| IBIS file stm32l4p5_4q5_ufqfpn48.ibs
[IBIS ver]   4.2
[File name]  stm32l4p5_4q5_ufqfpn48.ibs
[File Rev]   1.0
[Date]   26-12-2019
[Source]   Data Created at STMicroelectronics
[Notes]   File originated from ELDO simulations.
[Disclaimer] This information is for modeling purpose only and is
   not guaranted.
   The information is subject to change without notice.
[Copyright]  Copyright 2019 STMicroelectronics Inc.
|   Component stm32l4p5_4q5_ufqfpn48
[Component] stm32l4p5_4q5_ufqfpn48
[Manufacturer] STMicroelectronics
[Package]
| variable   typ   min   max
R_pkg  0  NA  NA
L_pkg  0  NA  NA
C_pkg  0  NA  NA
[Pin]   signal_name   model_name R_pin L_pin C_pin
1 VBAT POWER
2 PC13 io8prog2m25m50m120m_sudq_ft
3 PC14-OSC32_IN io8prog2m25m50m120m_sudq_ft
4 PC15-OSC32_OUT io8prog2m25m50m120m_sudq_ft
5 PH0-OSC_IN io8prog2m25m50m120m_sudq_ft
6 PH1-OSC_OUT io8prog2m25m50m120m_sudq_ft
7 NRST ioreset_ft_v33
8 VSSA GND
9 VDDA POWER
10 PA0 io8prog2m25m50m120m_sudq_ft
11 PA1 io8prog2m25m50m120m_sudq_ft
12 PA2 io8prog2m25m50m120m_sudq_ft
13 PA3 io8prog2m25m50m120m_sudq_ft
14 PA4 io8prog2m25m50m120m_sudq_ft
15 PA5 io8prog2m25m50m120m_sudq_ft
16 PA6 io8prog2m25m50m120m_sudq_ft
17 PA7 io8prog2m25m50m120m_sudq_ft
18 PB0 io8prog2m25m50m120m_sudq_ft
19 PB1 io8prog2m25m50m120m_sudq_ft
20 PB2 io8prog2m25m50m120m_sudq_ft
21 PB10 io8prog2m25m50m120m_sudq_i2c_ft
22 PB11 io8prog2m25m50m120m_sudq_i2c_ft
23 VSS GND
24 VDD POWER
25 PB12 io8w_swp_lcd4_ft
26 PB13 io8prog2m25m50m120m_sudq_i2c_ft
27 PB14 io8prog2m25m50m120m_sudq_i2c_ft
28 PB15 io8prog2m25m50m120m_sudq_ft
29 PA8 io8prog2m25m50m120m_sudq_ft
30 PA9 POWER
31 PA10 io8usb_id_otg20_lcd4_ft_ms
32 PA11 io8usblsfs_otg2
33 PA12 io8usblsfs_otg2
34 PA13 io8prog2m25m50m120m_sudq_ft
35 VSS GND
36 VDDUSB POWER
37 PA14 io8prog2m25m50m120m_sudq_ft
38 PA15 io8prog2m25m50m120m_sudq_ft
39 PB3 io8prog2m25m50m120m_sudq_ft
40 PB4 io8prog2m25m50m120m_sudq_ft
41 PB5 io8prog2m25m50m120m_sudq_ft
42 PB6 io8prog2m25m50m120m_sudq_i2c_ft
43 PB7 io8prog2m25m50m120m_sudq_i2c_ft
44 PH3-BOOT0 io8prog2m25m50m120m_sudq_ft
45 PB8 io8prog2m25m50m120m_sudq_i2c_ft
46 PB9 io8prog2m25m50m120m_sudq_i2c_ft
47 VSS GND
48 VDD POWER
[Model Selector] io8prog2m25m50m120m_sudq_ft
iols8p_sudq_ft_pd_lv  "IO low speed, PD=40kOhm - 1P8V"
iols8p_sudq_ft_pu_lv  "IO low speed, PU=40kOhm - 1P8V"
iols8p_sudq_ft_lv  "IO low speed - 1P8V"
iols8p_sudq_ft_pd  "IO low speed, PD=40kOhm - 3P3V"
iols8p_sudq_ft_pu  "IO low speed, PU=40kOhm - 3P3V"
iols8p_sudq_ft  "IO low speed - 3P3V"
iofs8p_sudq_ft_pd_lv  "IO full speed, PD=40kOhm - 1P8V"
iofs8p_sudq_ft_pu_lv  "IO full speed, PU=40kOhm - 1P8V"
iofs8p_sudq_ft_lv  "IO full speed - 1P8V"
iofs8p_sudq_ft_pd  "IO full speed, PD=40kOhm - 3P3V"
iofs8p_sudq_ft_pu  "IO full speed, PU=40kOhm - 3P3V"
iofs8p_sudq_ft  "IO full speed - 3P3V"
ioms8p_sudq_ft_pd_lv  "IO medium speed, PD=40kOhm - 1P8V"
ioms8p_sudq_ft_pu_lv  "IO medium speed, PU=40kOhm - 1P8V"
ioms8p_sudq_ft_lv  "IO medium speed - 1P8V"
ioms8p_sudq_ft_pd  "IO medium speed, PD=40kOhm - 3P3V"
ioms8p_sudq_ft_pu  "IO medium speed, PU=40kOhm - 3P3V"
ioms8p_sudq_ft  "IO medium speed - 3P3V"
iohs8p_sudq_ft_pd_lv  "IO high speed, PD=40kOhm - 1P8V"
iohs8p_sudq_ft_pu_lv  "IO high speed, PU=40kOhm - 1P8V"
iohs8p_sudq_ft_lv  "IO high speed - 1P8V"
iohs8p_sudq_ft_pd  "IO high speed, PD=40kOhm - 3P3V"
iohs8p_sudq_ft_pu  "IO high speed, PU=40kOhm - 3P3V"
iohs8p_sudq_ft  "IO high speed - 3P3V"
[Model Selector] io8prog2m25m50m120m_sudq_i2c_ft
io8prog_1v8_i2c_pd  "5V Tol GPIO 1.8V range i2c functionality with pull down"
io8prog_1v8_i2c_pu  "5V Tol GPIO 1.8V range i2c functionality with pull up"
io8prog_1v8_i2c  "5V Tol GPIO 1.8V range i2c functionality"
io8prog_3v3_i2c_pd  "5V Tol GPIO 3.3V range i2c functionality with pull down"
io8prog_3v3_i2c_pu  "5V Tol GPIO 3.3V range i2c functionality with pull up"
io8prog_3v3_i2c  "5V Tol GPIO 3.3V range i2c functionality"
iols8p_sudq_ft_pd_lv  "IO low speed, PD=40kOhm - 1P8V"
iols8p_sudq_ft_pu_lv  "IO low speed, PU=40kOhm - 1P8V"
iols8p_sudq_ft_lv  "IO low speed - 1P8V"
iols8p_sudq_ft_pd  "IO low speed, PD=40kOhm - 3P3V"
iols8p_sudq_ft_pu  "IO low speed, PU=40kOhm - 3P3V"
iols8p_sudq_ft  "IO low speed - 3P3V"
iofs8p_sudq_ft_pd_lv  "IO full speed, PD=40kOhm - 1P8V"
iofs8p_sudq_ft_pu_lv  "IO full speed, PU=40kOhm - 1P8V"
iofs8p_sudq_ft_lv  "IO full speed - 1P8V"
iofs8p_sudq_ft_pd  "IO full speed, PD=40kOhm - 3P3V"
iofs8p_sudq_ft_pu  "IO full speed, PU=40kOhm - 3P3V"
iofs8p_sudq_ft  "IO full speed - 3P3V"
ioms8p_sudq_ft_pd_lv  "IO medium speed, PD=40kOhm - 1P8V"
ioms8p_sudq_ft_pu_lv  "IO medium speed, PU=40kOhm - 1P8V"
ioms8p_sudq_ft_lv  "IO medium speed - 1P8V"
ioms8p_sudq_ft_pd  "IO medium speed, PD=40kOhm - 3P3V"
ioms8p_sudq_ft_pu  "IO medium speed, PU=40kOhm - 3P3V"
ioms8p_sudq_ft  "IO medium speed - 3P3V"
iohs8p_sudq_ft_pd_lv  "IO high speed, PD=40kOhm - 1P8V"
iohs8p_sudq_ft_pu_lv  "IO high speed, PU=40kOhm - 1P8V"
iohs8p_sudq_ft_lv  "IO high speed - 1P8V"
iohs8p_sudq_ft_pd  "IO high speed, PD=40kOhm - 3P3V"
iohs8p_sudq_ft_pu  "IO high speed, PU=40kOhm - 3P3V"
iohs8p_sudq_ft  "IO high speed - 3P3V"
[Model Selector] io8w_swp_lcd4_ft
io8w_swp_classc  "Class C swp functionality"
io8w_swp_classb  "Class B swp functionality"
io8lsw_1v8_pd  "GPIO 1.8V range with pd io low speed"
io8lsw_1v8_pu  "GPIO 1.8V range with pu io low speed"
io8lsw_1v8  "GPIO 1.8V range io low speed"
io8lsw_3v3_pd  "GPIO 3.3V range with pd io low speed"
io8lsw_3v3_pu  "GPIO 3.3V range with pu io low speed"
io8lsw_3v3  "GPIO 3.3V range io low speed"
io8fsw_1v8_pd  "GPIO 1.8V range with pd io full speed"
io8fsw_1v8_pu  "GPIO 1.8V range with pu io full speed"
io8fsw_1v8  "GPIO 1.8V range io full speed"
io8fsw_3v3_pd  "GPIO 3.3V range with pd io full speed"
io8fsw_3v3_pu  "GPIO 3.3V range with pu io full speed"
io8fsw_3v3  "GPIO 3.3V range io full speed"
io8msw_1v8_pd  "GPIO 1.8V range with pd io medium speed"
io8msw_1v8_pu  "GPIO 1.8V range with pu io medium speed"
io8msw_1v8  "GPIO 1.8V range io medium speed"
io8msw_3v3_pd  "GPIO 3.3V range with pd io medium speed"
io8msw_3v3_pu  "GPIO 3.3V range with pu io medium speed"
io8msw_3v3  "GPIO 3.3V range io medium speed"
io8hsw_1v8_pd  "GPIO 1.8V range with pd io high speed"
io8hsw_1v8_pu  "GPIO 1.8V range with pu io high speed"
io8hsw_1v8  "GPIO 1.8V range io high speed"
io8hsw_3v3_pd  "GPIO 3.3V range with pd io high speed"
io8hsw_3v3_pu  "GPIO 3.3V range with pu io high speed"
io8hsw_3v3  "GPIO 3.3V range io high speed"
[Model Selector] io8usblsfs_otg2
usb_ls_pd  "USB Low Speed mode - Pull Down"
usb_ls_pu2  "USB Low Speed mode - Pull up 2"
usb_ls_pu  "USB Low Speed mode - Pull up"
usb_fs  "USB Low Speed mode"
usb_fs_pd  "USB Full Speed mode - Pull Down"
usb_fs_pu2  "USB Full Speed mode - Pull up 2"
usb_fs_pu  "USB Full Speed mode - Pull up"
[Model Selector] io8usb_id_otg20_lcd4_ft_ms
io8usbid_1v8_id_pu  "ID 1V8 range with pull up"
io8usbid_3v3_id_pu  "ID 3V3 range with pull up"
io8usbid_1v8_id  "ID 1V8 range"
io8usbid_3v3_id  "ID 3V3 range"
io8lsusbid_1v8_pd  "GPIO 1.8V range with pd io low speed"
io8lsusbid_1v8_pu  "GPIO 1.8V range with pu io low speed"
io8lsusbid_1v8  "GPIO 1.8V range io low speed"
io8lsusbid_3v3_pd  "GPIO 3.3V range with pd io low speed"
io8lsusbid_3v3_pu  "GPIO 3.3V range with pu io low speed"
io8lsusbid_3v3  "GPIO 3.3V range io low speed"
io8fsusbid_1v8_pd  "GPIO 1.8V range with pd io full speed"
io8fsusbid_1v8_pu  "GPIO 1.8V range with pu io full speed"
io8fsusbid_1v8  "GPIO 1.8V range io full speed"
io8fsusbid_3v3_pd  "GPIO 3.3V range with pd io full speed"
io8fsusbid_3v3_pu  "GPIO 3.3V range with pu io full speed"
io8fsusbid_3v3  "GPIO 3.3V range io full speed"
io8msusbid_1v8_pd  "GPIO 1.8V range with pd io medium speed"
io8msusbid_1v8_pu  "GPIO 1.8V range with pu io medium speed"
io8msusbid_1v8  "GPIO 1.8V range io medium speed"
io8msusbid_3v3_pd  "GPIO 3.3V range with pd io medium speed"
io8msusbid_3v3_pu  "GPIO 3.3V range with pu io medium speed"
io8msusbid_3v3  "GPIO 3.3V range io medium speed"
io8hsusbid_1v8_pd  "GPIO 1.8V range with pd io high speed"
io8hsusbid_1v8_pu  "GPIO 1.8V range with pu io high speed"
io8hsusbid_1v8  "GPIO 1.8V range io high speed"
io8hsusbid_3v3_pd  "GPIO 3.3V range with pd io high speed"
io8hsusbid_3v3_pu  "GPIO 3.3V range with pu io high speed"
io8hsusbid_3v3  "GPIO 3.3V range io high speed"
[Model Selector] ioreset_ft_v33
ioreset_1v2_pu  "RESET 1.2V range with PU"
ioreset_1v2  "RESET 1.2V range"
ioreset_1v8_pu  "RESET 1.8V range with PU"
ioreset_1v8  "RESET 1.8V range"
ioreset_3v3_pu  "RESET 3.3V range with PU"
ioreset_3v3  "RESET 3.3V range"
| Models and submodels in the file (97): iols8p_sudq_ft_pd_lv (I/O), iols8p_sudq_ft_pu_lv (I/O), iols8p_sudq_ft_lv (I/O), iols8p_sudq_ft_pd (I/O), iols8p_sudq_ft_pu (I/O), iols8p_sudq_ft (I/O), iofs8p_sudq_ft_pd_lv (I/O), iofs8p_sudq_ft_pu_lv (I/O), iofs8p_sudq_ft_lv (I/O), iofs8p_sudq_ft_pd (I/O), iofs8p_sudq_ft_pu (I/O), iofs8p_sudq_ft (I/O), ioms8p_sudq_ft_pd_lv (I/O), ioms8p_sudq_ft_pu_lv (I/O), ioms8p_sudq_ft_lv (I/O), ioms8p_sudq_ft_pd (I/O), ioms8p_sudq_ft_pu (I/O), ioms8p_sudq_ft (I/O), iohs8p_sudq_ft_pd_lv (I/O), iohs8p_sudq_ft_pu_lv (I/O), iohs8p_sudq_ft_lv (I/O), iohs8p_sudq_ft_pd (I/O), iohs8p_sudq_ft_pu (I/O), iohs8p_sudq_ft (I/O), io8prog_1v8_i2c_pd (I/O_open_drain), io8prog_1v8_i2c_pu (I/O_open_drain), io8prog_1v8_i2c (I/O_open_drain), io8prog_3v3_i2c_pd (I/O_open_drain), io8prog_3v3_i2c_pu (I/O_open_drain), io8prog_3v3_i2c (I/O_open_drain), io8w_swp_classc (I/O), io8w_swp_classb (I/O), io8lsw_1v8_pd (I/O), io8lsw_1v8_pu (I/O), io8lsw_1v8 (I/O), io8lsw_3v3_pd (I/O), io8lsw_3v3_pu (I/O), io8lsw_3v3 (I/O), io8fsw_1v8_pd (I/O), io8fsw_1v8_pu (I/O), io8fsw_1v8 (I/O), io8fsw_3v3_pd (I/O), io8fsw_3v3_pu (I/O), io8fsw_3v3 (I/O), io8msw_1v8_pd (I/O), io8msw_1v8_pu (I/O), io8msw_1v8 (I/O), io8msw_3v3_pd (I/O), io8msw_3v3_pu (I/O), io8msw_3v3 (I/O), io8hsw_1v8_pd (I/O), io8hsw_1v8_pu (I/O), io8hsw_1v8 (I/O), io8hsw_3v3_pd (I/O), io8hsw_3v3_pu (I/O), io8hsw_3v3 (I/O), usb_ls_pd (I/O), usb_ls_pu2 (I/O), usb_ls_pu (I/O), usb_fs (I/O), usb_fs_pd (I/O), usb_fs_pu2 (I/O), usb_fs_pu (I/O), io8usbid_1v8_id_pu (Input), io8usbid_3v3_id_pu (Input), io8usbid_1v8_id (Input), io8usbid_3v3_id (Input), io8lsusbid_1v8_pd (I/O), io8lsusbid_1v8_pu (I/O), io8lsusbid_1v8 (I/O), io8lsusbid_3v3_pd (I/O), io8lsusbid_3v3_pu (I/O), io8lsusbid_3v3 (I/O), io8fsusbid_1v8_pd (I/O), io8fsusbid_1v8_pu (I/O), io8fsusbid_1v8 (I/O), io8fsusbid_3v3_pd (I/O), io8fsusbid_3v3_pu (I/O), io8fsusbid_3v3 (I/O), io8msusbid_1v8_pd (I/O)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
